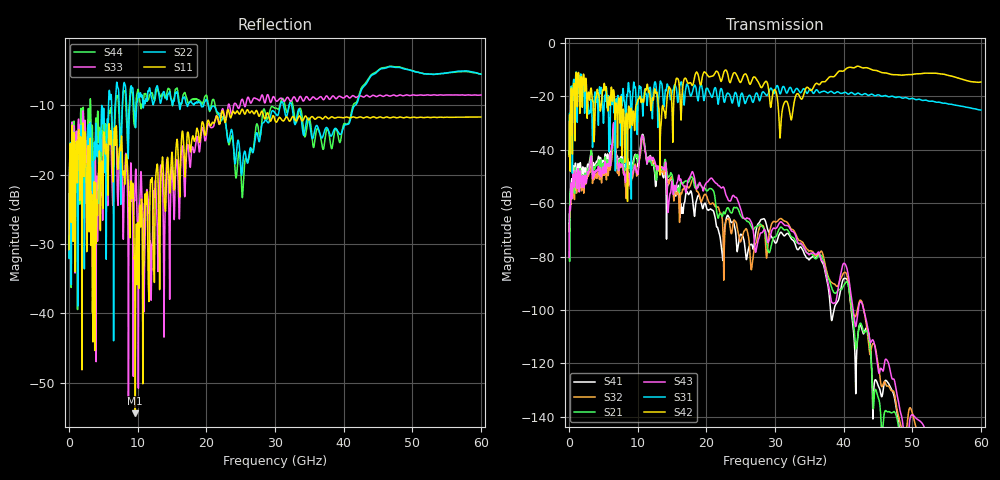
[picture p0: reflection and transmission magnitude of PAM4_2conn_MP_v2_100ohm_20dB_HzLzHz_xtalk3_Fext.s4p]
! Info: Touchstone file created by Circ.  Input file=FAB50GbE_2conn_Midplane_Examax_Topo2_v2_100ohm_20dB_HzLzHz.circ
# Hz S RI R 50
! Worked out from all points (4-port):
!   6000 points, 10 MHz to 60 GHz, reference 50 ohm
!   strongest paths, dB at 10 MHz, 15.01 GHz, 30.01 GHz, 45.01 GHz, 60 GHz:
!     S42: -42.5, -25.2, -17.5, -10.5, -14.7
!     S31: -41.8, -18.9, -18.0, -19.4, -25.1
!     S43: -80.3, -51.8, -69.5, -121.8, -160.5
!     S21: -64.1, -49.3, -72.7, -132.5, -166.1
!     S32: -68.2, -50.2, -67.1, -120.1, -163.2
!     S41: -67.6, -50.3, -74.8, -128.2, -180.9
!   lowest |S11| = -54.4 dB at 9.65 GHz (marker M1), VSWR 1.00, Z = 50.1 - j0.156 ohm
!   |S11| at or under -10 dB: start of sweep to end of sweep
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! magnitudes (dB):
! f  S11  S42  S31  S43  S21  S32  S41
! 10 MHz  -30.8  -42.5  -41.8  -80.3  -64.1  -68.2  -67.6
! 1.22 GHz  -20.8  -22.9  -22.4  -49.9  -49.4  -51.1  -47.1
! 6.44 GHz  -20.3  -17.7  -19.7  -30.9  -33.4  -35.6  -31.4
! 9.65 GHz  -54.4  -26.5  -16.6  -46.8  -42.2  -45.4  -41.7
! 22.25 GHz  -11.0  -13.9  -17.5  -54.3  -64.8  -64.6  -77.4
! 27.26 GHz  -10.8  -13.4  -18.8  -77.7  -68.9  -74.9  -70.0
! 60 GHz  -11.7  -14.7  -25.1  -160.5  -166.1  -163.2  -180.9
